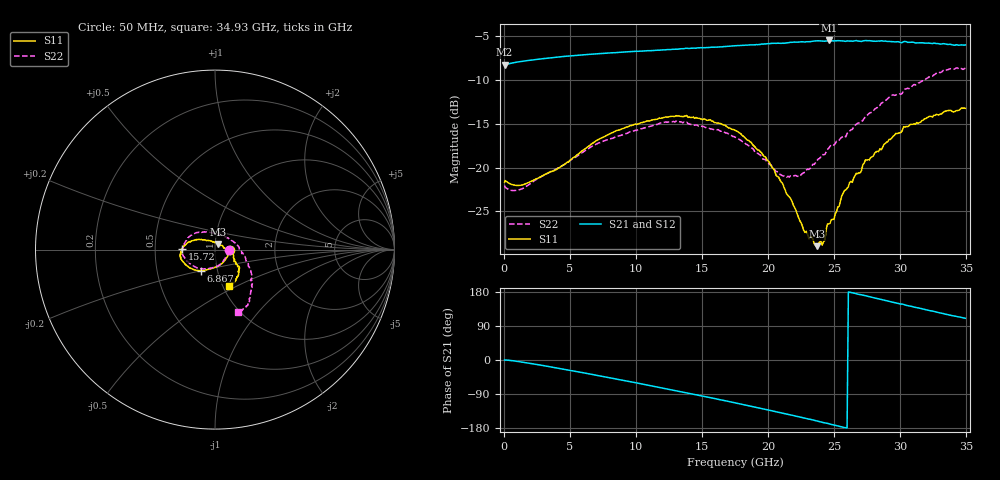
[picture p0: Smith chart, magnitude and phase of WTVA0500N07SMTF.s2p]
! 50 ohm 2-Port S-parameters measured by Modelithics Inc support@modelithics.com  Tampa, FL USA 813-866-6335 (February 2024)
! Smiths Interconnect,  5dB P/N: WTVA0500N07SMTF, Temperature: -25 C
! Board: 10 mil Rogers 4350B,Mounting Pad Dimensions: Length: 15 mils, Width: 25 mils, Gap: 40 mils.
# Hz S RI R 50
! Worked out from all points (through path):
!   352 points, 50 MHz to 34.93 GHz, reference 50 ohm
!   highest |S21| = -5.47 dB at 24.58 GHz (marker M1); lowest = -8.3 dB at 50 MHz (marker M2)
!   group delay of S21, straight-line fit = 20.4 ps
!   lowest |S11| = -29.0 dB at 23.68 GHz (marker M3), VSWR 1.07, Z = 51.5 + j3.29 ohm
!   |S11| at or under -10 dB: start of sweep to end of sweep
!   |S22| runs from -22.6 to -8.6 dB; largest |S21 - S12| = 0.0049
!   S11 on the Smith chart (normalised r, x): 50 MHz: 1.18, -0.01; 6.867 GHz: 0.84, -0.20; 15.72 GHz: 0.69, +0.00; 34.93 GHz: 1.07, -0.46
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5e7  0.0826 -0.00293  0.3867 0.000445  0.3864 0.000383  0.0789 -0.00263
1.2945e9  0.0612 -0.0505  0.4024 -0.0364  0.4021 -0.0365  0.0542 -0.0522
5.8715e9  -0.0498 -0.1135  0.3697 -0.2388  0.3693 -0.2389  -0.0558 -0.1073
6.8665e9  -0.0768 -0.1174  0.3447 -0.2826  0.3441 -0.2826  -0.0823 -0.1066
1.1742e10  -0.1793 -0.068  0.1436 -0.446  0.1424 -0.446  -0.1741 -0.0397
1.5722e10  -0.1843 0.00327  -0.0859 -0.4801  -0.0871 -0.4796  -0.1568 0.0553
1.7513e10  -0.1599 0.0316  -0.1962 -0.4563  -0.1972 -0.4556  -0.1212 0.087
1.98015e10  -0.1 0.0568  -0.3296 -0.3879  -0.3297 -0.3875  -0.0493 0.0994
2.13935e10  -0.0488 0.0513  -0.4085 -0.3148  -0.4091 -0.3135  0.0135 0.087
2.2687e10  -0.0119 0.0421  -0.4655 -0.2381  -0.4657 -0.2369  0.0635 0.0686
2.33835e10  0.00937 0.0379  -0.4901 -0.1959  -0.4901 -0.1948  0.089 0.055
2.3682e10  0.0157 0.0319  -0.5004 -0.1744  -0.5003 -0.1735  0.0983 0.0476
2.4279e10  0.0303 0.0233  -0.5111 -0.1297  -0.5112 -0.1284  0.1152 0.0284
2.4478e10  0.0422 0.022  -0.5164 -0.1181  -0.5165 -0.1169  0.1241 0.0251
2.45775e10  0.0451 0.0154  -0.5214 -0.1098  -0.5214 -0.1083  0.1273 0.0213
2.49755e10  0.0499 0.00883  -0.5237 -0.0779  -0.5237 -0.0765  0.1345 0.0043
2.57715e10  0.0739 -0.00361  -0.528 -0.0163  -0.5277 -0.0153  0.1504 -0.0214
2.73635e10  0.1046 -0.0362  -0.5231 0.0986  -0.5225 0.1002  0.181 -0.0718
2.91545e10  0.1201 -0.0812  -0.475 0.2265  -0.4737 0.2282  0.2063 -0.1448
3.0249e10  0.137 -0.1029  -0.4373 0.2898  -0.4358 0.2914  0.2093 -0.1802
3.2836e10  0.1169 -0.1625  -0.2975 0.4159  -0.2972 0.4158  0.1883 -0.2963
3.49255e10  0.0785 -0.2035  -0.1726 0.4715  -0.1688 0.4725  0.1262 -0.3483
